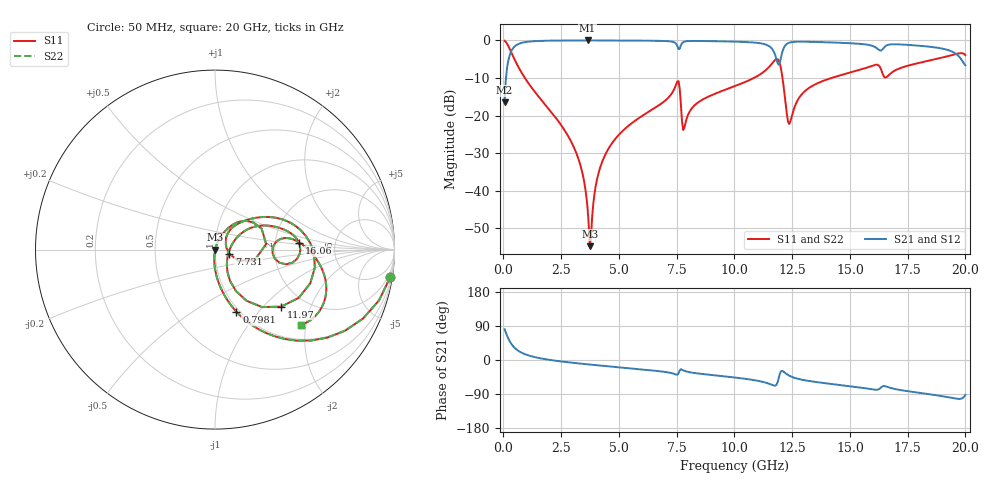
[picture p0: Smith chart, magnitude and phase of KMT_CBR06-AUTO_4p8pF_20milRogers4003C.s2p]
! Data measured by Modelithics Inc. support@modelithics.com 813-866-6335
! KEMET CBR06-AUTO 4.8pF, Pad Width= 0.851mm, Pad Length= 0.64mm, Pad Gap= 0.62mm, 20mil Rogers 4003C substrate Data, January 2022
# hz S ma R 50
! 2 Port Network Data from SP1.SP block
! freq  magS11  angS11  magS21  angS21  magS12  angS12  magS22  angS22
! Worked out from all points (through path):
!   401 points, 50 MHz to 20 GHz, reference 50 ohm
!   highest |S21| = -0.02 dB at 3.641 GHz (marker M1); lowest = -16.5 dB at 50 MHz (marker M2)
!   group delay of S21, straight-line fit = 15.9 ps
!   lowest |S11| = -54.7 dB at 3.741 GHz (marker M3), VSWR 1.00, Z = 50.2 - j0.104 ohm
!   |S11| at or under -10 dB: 928.4 MHz to 10.84 GHz (9.91 GHz wide, 168 % of centre); 12.08 GHz to 14.2 GHz (2.121 GHz wide, 16.1 % of centre)
!   |S22| runs from -54.7 to -0.1 dB; largest |S21 - S12| = 0
!   S11 on the Smith chart (normalised r, x): 50 MHz: 1, -13; 798.1 MHz: 0.97, -0.77; 7.731 GHz: 1.17, -0.06; 11.97 GHz: 1.53, -1.27; 16.06 GHz: 2.74, +0.26; 20 GHz: 1.33, -1.89
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5e7  0.9886 -8.8  0.1503 81.2  0.1503 81.2  0.9886 -8.8
2.99375e8  0.7372 -43.4  0.6749 46.5  0.6749 46.5  0.7372 -43.4
7.98125e8  0.3666 -70.9  0.9294 18.9  0.9294 18.9  0.3666 -70.9
2.693375e9  0.06056 -93.8  0.9966 -5.2  0.9966 -5.2  0.06056 -93.8
3.391625e9  0.01861 -94.9  0.9981 -9.9  0.9981 -9.9  0.01861 -94.9
3.641e9  0.005886 -84.9  0.9982 -11.4  0.9982 -11.4  0.005886 -84.9
3.74075e9  0.001834 -34.4  0.9982 -12.0  0.9982 -12.0  0.001834 -34.4
4.089875e9  0.01596 69.5  0.998 -14.1  0.998 -14.1  0.01596 69.5
4.53875e9  0.03595 70.3  0.9973 -16.7  0.9973 -16.7  0.03595 70.3
6.73325e9  0.1374 58.8  0.9863 -29.5  0.9863 -29.5  0.1374 58.8
7.53125e9  0.2849 24.1  0.8374 -38.9  0.8374 -38.9  0.2849 24.1
7.73075e9  0.08365 -16.5  0.917 -25.5  0.917 -25.5  0.08365 -16.5
1.0025e10  0.2472 42.4  0.9629 -46.3  0.9629 -46.3  0.2472 42.4
1.147138e10  0.4347 21.1  0.8499 -62.1  0.8499 -62.1  0.4347 21.1
1.177062e10  0.5524 -2.5  0.6315 -67.4  0.6315 -67.4  0.5524 -2.5
1.197012e10  0.4867 -40.8  0.514 -35.4  0.514 -35.4  0.4867 -40.8
1.236912e10  0.07732 -14.6  0.9299 -41.2  0.9299 -41.2  0.07732 -14.6
1.336662e10  0.2477 30.5  0.956 -56.6  0.956 -56.6  0.2477 30.5
1.605988e10  0.4698 4.5  0.8253 -78.3  0.8253 -78.3  0.4698 4.5
1.670825e10  0.3513 8.0  0.8809 -72.8  0.8809 -72.8  0.3513 8.0
1.890275e10  0.5811 -7.1  0.7877 -94.5  0.7877 -94.5  0.5811 -7.1
2e10  0.6384 -41.1  0.4655 -92.0  0.4655 -92.0  0.6384 -41.1
